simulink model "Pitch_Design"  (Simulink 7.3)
settings: Solver=ode45  StartTime=0.0  StopTime=10.0  RelTol=1e-3
undefined symbols (not defined in the file or in its folder): Ap, Bp, Cp, Dp

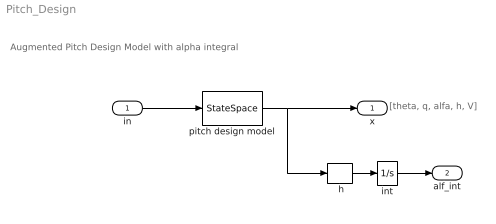
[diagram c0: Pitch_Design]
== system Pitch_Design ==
  note: Augmented Pitch Design Model with alpha integral
  note: [theta, q, alfa, h, V]
  in : Inport  OutDataType=sfix(16)  OutScaling=2^0
  " h" : Selector  InputPortWidth=5  IndexOptions=Index vector (dialog)  Indices=[3]  OutputSizes=1
  int : Integrator
  pitch design model : StateSpace  A=Ap  B=Bp  C=Cp  D=Dp
  x : Outport  OutDataType=sfix(16)  OutScaling=2^0
  alf_int : Outport  Port=2  OutDataType=sfix(16)  OutScaling=2^0
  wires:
  in/1 -> pitch design model/1
  pitch design model/1 -> x/1, " h"/1
  " h"/1 -> int/1
  int/1 -> alf_int/1
